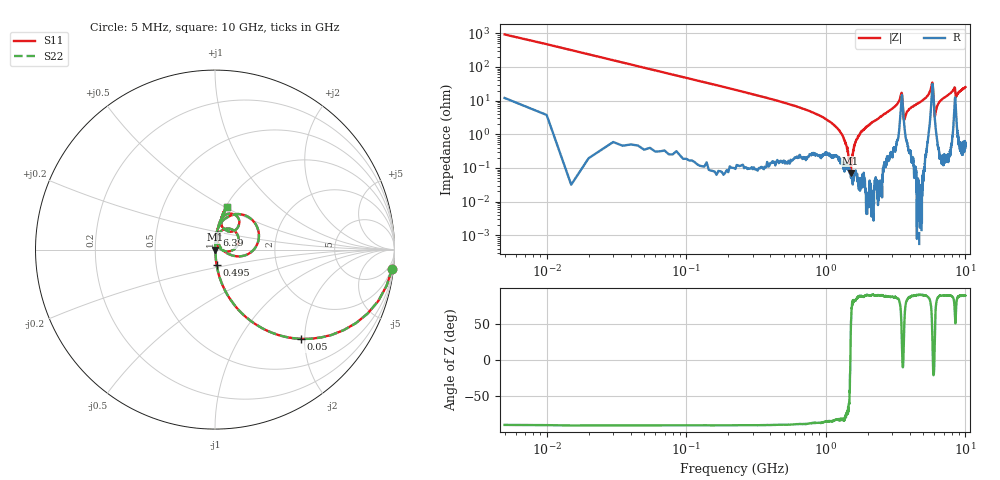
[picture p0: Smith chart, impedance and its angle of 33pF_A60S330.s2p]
! Amotech Co.,Ltd.
! http://www.amotech.co.kr/
! Part Number: A60S330
! These Parameters are Measured in Series Mode Connection
! Operation Temp=25[degC], DC Bias Voltage=0[V]
! Freq. Start=5[MHz] Stop=10[GHz], 2000[Steps]
! Date: Monday, July 13, 2020, 01:41:22
# GHZ S RI R 50.000000
!Freq.(Hz) S11(Real) S11(Imag) S21(Real) S21(Imag) S12(Real) S12(Imag) S22(Real) S22(Imag)
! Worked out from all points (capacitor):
!   2000 points, 5 MHz to 10 GHz, reference 50 ohm
!   read as one part in series: C = 33.3 pF near 55 MHz
!   lowest |Z| = 70.4 mohm at 1.505 GHz (marker M1)
!   series resonance near 1.499 GHz, so ESL is about 340 pH
!   S11 on the Smith chart (normalised r, x): 5 MHz: 1, -18; 50 MHz: 1.01, -1.91; 495 MHz: 1.00, -0.18; 6.39 GHz: 1.01, +0.16; 10 GHz: 1.01, +0.51
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0.005  0.987 -0.1067  0.013 0.1067  0.013 0.1067  0.987 -0.1067
0.05  0.4766 -0.4976  0.5234 0.4976  0.5234 0.4976  0.4766 -0.4976
0.155  0.0868 -0.2802  0.9132 0.2802  0.9132 0.2802  0.0868 -0.2802
0.495  0.00936 -0.0879  0.9906 0.0879  0.9906 0.0879  0.00936 -0.0879
1.24  0.00197 -0.0133  0.998 0.0133  0.998 0.0133  0.00197 -0.0133
1.375  0.00116 -0.00569  0.9988 0.00569  0.9988 0.00569  0.00116 -0.00569
1.505  0.000664 0.000232  0.9993 -0.000232  0.9993 -0.000232  0.000664 0.000232
1.675  0.000705 0.00736  0.9993 -0.00736  0.9993 -0.00736  0.000705 0.00736
2.13  0.000524 0.0221  0.9995 -0.0221  0.9995 -0.0221  0.000524 0.0221
3.34  0.0199 0.0916  0.9801 -0.0916  0.9801 -0.0916  0.0199 0.0916
3.49  0.1227 0.0876  0.8773 -0.0876  0.8773 -0.0876  0.1227 0.0876
3.655  0.017 0.0209  0.983 -0.0209  0.983 -0.0209  0.017 0.0209
3.97  0.00598 0.0565  0.994 -0.0565  0.994 -0.0565  0.00598 0.0565
5.005  0.0116 0.1053  0.9884 -0.1053  0.9884 -0.1053  0.0116 0.1053
5.775  0.2214 0.1491  0.7786 -0.1491  0.7786 -0.1491  0.2214 0.1491
5.85  0.2047 -0.0111  0.7953 0.0111  0.7953 0.0111  0.2047 -0.0111
6.035  0.0295 0.0147  0.9705 -0.0147  0.9705 -0.0147  0.0295 0.0147
6.39  0.0103 0.0793  0.9897 -0.0793  0.9897 -0.0793  0.0103 0.0793
6.67  0.0122 0.1001  0.9878 -0.1001  0.9878 -0.1001  0.0122 0.1001
8.335  0.0945 0.1999  0.9055 -0.1999  0.9055 -0.1999  0.0945 0.1999
8.565  0.058 0.1095  0.942 -0.1095  0.942 -0.1095  0.058 0.1095
10  0.0648 0.2366  0.9352 -0.2366  0.9352 -0.2366  0.0648 0.2366
